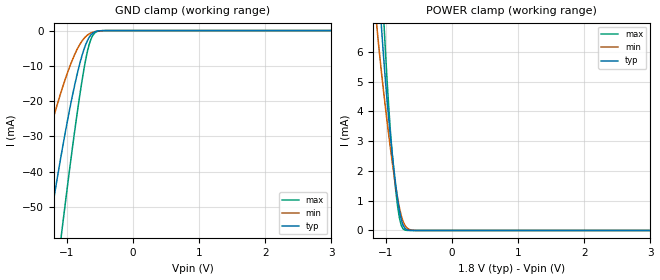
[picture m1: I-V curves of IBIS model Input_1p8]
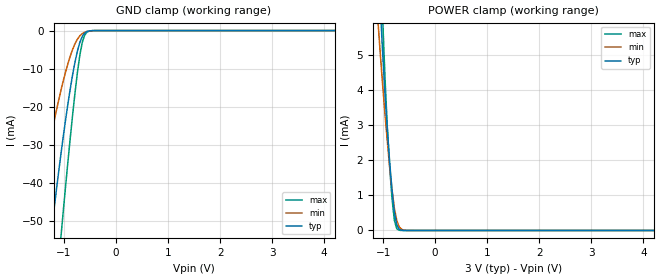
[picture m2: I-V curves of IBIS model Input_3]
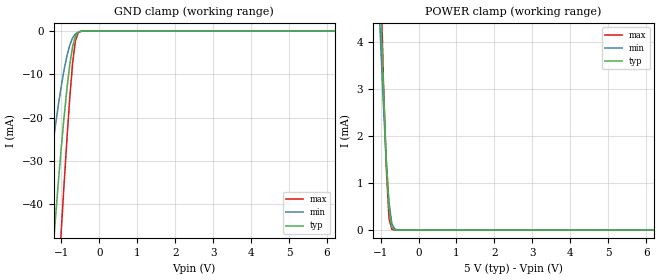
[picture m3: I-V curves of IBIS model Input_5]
|Texas Instruments Incorporated
|18-bit, Single Channgel, Low-Noise, Voltage-Output
|DIGITAL-TO-ANALOG CONVERTER
| Marketing part#   Voltage Range   Package-type   #pins
|DAC9881SBRGER   1.7V - 5V   VQFN   24-pin RGE
|DAC9881SBRGERG4   1.7V - 5V   VQFN   24-pin RGE
|DAC9881SBRGET   1.7V - 5V   VQFN   24-pin RGE
|DAC9881SBRGETG4   1.7V - 5V   VQFN   24-pin RGE
|DAC9881SRGER   1.7V - 5V   VQFN   24-pin RGE
|DAC9881SRGERG4   1.7V - 5V   VQFN   24-pin RGE
|DAC9881SRGET   1.7V - 5V   VQFN   24-pin RGE
|DAC9881SRGETG4   1.7V - 5V   VQFN   24-pin RGE
[IBIS Ver]   4.0
[File name]   dac9881a.ibs
[File Rev]   1.0
[Date]   07/08/2009
[Source]   Texas Instruments Incorporated.
   Analog-eLab, HPA
   12500 TI Blvd
   Dallas, TX -75243
   For Support e-mail: elab_ibis@list.ti.com
[Notes]   Revision History:
   1.0: 07/08/2009
   - Initial Model generated from simulations in TISPICED
   - Model not matched to measurements
   - Ignore warnings related to ccomp min max values, these are
   as per simulations in TISPICED, part uses BJT devices
[Disclaimer]
 This product is designed as an aid for customers of Texas Instruments.
 No warranties, either expressed or implied, with respect to this third
 party software (if any) or with respect to its fitness for any
 particular purpose is claimed by Texas Instruments or the author. The
 software (if any) is provided solely on an "as is" basis. The entire
 risk as to its quality and performance is with the customer
[Copyright] (C) Copyright 2009 Texas Instruments Incorporated.
   All rights reserved.
|   DAC9881A
[Component]   DAC9881A
[Manufacturer]  Texas Instruments Incorporated
[Package]   |24-pin RGE, VQFN 4mm X 4mm
|   typ   min   max
R_pkg   71.83m   62.81m   80.84m
L_pkg   1.169nH   1.006nH   1.332nH
C_pkg   0.103pF   0.094pF   0.112pF
[Pin]   signal_name   model_name   R_pin   L_pin   C_pin
   1   SCLK   Input   0.07599  1.23841nH   0.10623pF
   2   SDI   Input   0.07182  1.16214nH   0.10564pF
   3   LDAC#   Input   0.07043  1.13785nH   0.10439pF
   4   AGND   GND   0.03576  0.79035nH   0.14259pF
   5   AVDD   POWER   0.07196  1.16684nH   0.10654pF
   6   VREFLS   NC   0.07706  1.26253nH   0.10829pF
   7   VREFHS   NC   0.07013  1.13811nH   0.10024pF
   8   VOUT   NC   0.06281  1.00570nH   0.09441pF
   9   RFB   NC   0.06661  1.07325nH   0.10032pF
   10   VREFLF   NC   0.03298  0.69750nH   0.14107pF
   11   VREFHF   NC   0.03275  0.70664nH   0.14010pF
   12   NC   NC   0.07739  1.27043nH   0.11226pF
   13   NC   NC   0.08084  1.33221nH   0.11195pF
   14   RSTSEL   Input   0.07657  1.25184nH   0.11077pF
   15   GAIN   Input   0.07212  1.16965nH   0.10607pF
   16   USB_BTC#   Input   0.07043  1.13795nH   0.10403pF
   17   RST#   Input   0.07196  1.16454nH   0.10595pF
   18   PDN   Input   0.07653  1.24823nH   0.10633pF
   19   CS#   Input   0.07679  1.25161nH   0.10889pF
   20   SDOSEL   Input   0.06908  1.10924nH   0.10603pF
   21   AVDD   POWER   0.06763  1.08295nH   0.10070pF
   22   DGND   GND   0.06770  1.08415nH   0.09968pF
   23   SDO   Output   0.06834  1.09604nH   0.10367pF
   24   IOVDD   POWER   0.07464  1.21210nH   0.10622pF
|   25   NC   NC   0.00089  0.24393nH  1.30974pF  ||mountpad
[Model Selector]   Input
Input_1p8   IOVDD varies between 1.7V - 2.0V, typ value being 1.8V
Input_3   IOVDD varies between 2.7V - 3.3V, typ value being 3.0V
Input_5   IOVDD varies between 4.5V - 5.5V, typ value being 5.0V
[Model Selector]   Output
Output_1p8   IOVDD varies between 1.7V - 2.0V, typ value being 1.8V
Output_3   IOVDD varies between 2.7V - 3.3V, typ value being 3.0V
Output_5   IOVDD varies between 4.5V - 5.5V, typ value being 5.0V
| Models and submodels in the file (6): Input_1p8 (Input), Input_3 (Input), Input_5 (Input), Output_1p8 (3-state), Output_3 (3-state), Output_5 (3-state)
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|   Input 1.8V IOVDD
[Model]   Input_1p8
Model_type   Input
|Signals
|Input Levels
Vinl = 0V
Vinh = 1.5V
|   typ   min   max
C_comp   3.032pF   3.426pF   2.439pF
[Model Spec]
Vinl   0V   -0.3V   0.3V
Vinh   1.9V   1.5V   2.3V
[Voltage Range]   1.8V   1.7V   2.0V
| Junction Temperature (Ambient temp is 25C typ, 85C min,  -40C max)
[Temperature Range]   27.0   105.0   -40.0
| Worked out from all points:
|   GND clamp passes 1 mA (typ) near -0.62 V on its own axis
|   POWER clamp passes 1 mA (typ) near -0.82 V on its own axis
[GND Clamp]
|   Voltage   I(typ)   I(min)   I(max)
-1.8V     -124.5mA   -72.43mA   -174.7mA
-1.61V    -99.18mA   -55.82mA   -143.3mA
-1.284V   -58.12mA   -30.4mA    -90.01mA
-1.257V   -54.89mA   -28.5mA    -85.65mA
-1.067V   -33.54mA   -16.32mA   -55.8mA
-931.7mV  -20.04mA   -9.093mA   -35.69mA
-823.1mV  -10.85mA   -4.6mA     -20.89mA
-741.7mV  -5.439mA   -2.278mA   -11.1mA
-660.3mV  -1.897mA   -933.9uA   -3.886mA
-578.9mV  -387.6uA   -321.7uA   -706.2uA
-470.4mV  -25.45uA   -52.46uA   -29.69uA
3.6V      0A         0A         0A
[POWER Clamp]
|   Voltage   I(typ)   I(min)   I(max)
-1.8V     36.64mA    28.31mA    45.65mA
-1.149V   9.666mA    7.122mA    12.38mA
-1.122V   8.678mA    6.481mA    11.09mA
-1.067V   6.82mA     5.306mA    8.583mA
-1.04V    5.967mA    4.76mA     7.384mA
-1.013V   5.177mA    4.233mA    6.238mA
-931.7mV  3.15mA     2.753mA    3.312mA
-850.3mV  1.504mA    1.451mA    1.307mA
-796mV    664.8uA    761.1uA    419.8uA
-714.6mV  74.74uA    176.1uA    16.51uA
-524.6mV  78.53nA    1.039uA    4.643nA
3.6V      0A         0A         0A
|   Input 3.0V IOVDD
[Model]   Input_3
Model_type   Input
Vinl = 0.15V
Vinh = 2.85V
|   typ   min   max
C_comp   2.779pF   3.181pF   2.237pF
[Model Spec]
Vinl   0.15V   -0.3V   0.6V
Vinh   2.85V   2.1V   3.6V
[Voltage Range]   3.000V   2.700V   3.300V
| Junction Temperature (Ambient temp is 25C typ, 105C min,  -40C max)
[Temperature Range]   27.0   105.0   -40.0
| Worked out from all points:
|   GND clamp passes 1 mA (typ) near -0.62 V on its own axis
|   POWER clamp passes 1 mA (typ) near -0.82 V on its own axis
[GND Clamp]
|   Voltage   I(typ)   I(min)   I(max)
-3V       -292.7mA   -193.9mA   -373.2mA
-1.598V   -97.6mA    -54.8mA    -141.3mA
-1.553V   -91.7mA    -51.04mA   -133.8mA
-1.236V   -52.41mA   -27.04mA   -82.27mA
-1.055V   -32.27mA   -15.62mA   -53.96mA
-1.01V    -27.62mA   -13.09mA   -47.15mA
-874.4mV  -14.97mA   -6.547mA   -27.69mA
-738.7mV  -5.271mA   -2.211mA   -10.78mA
-648.2mV  -1.554mA   -806.3uA   -3.158mA
-603mV    -656.4uA   -449.5uA   -1.26mA
-422.1mV  -6.58uA    -17.45uA   -5.716uA
6V        0A         0A         0A
[POWER Clamp]
|   Voltage   I(typ)   I(min)   I(max)
-3V       88.98mA    71.68mA    109mA
-1.101V   7.934mA    6.009mA    10.1mA
-1.055V   6.434mA    5.06mA     8.045mA
-1.01V    5.093mA    4.176mA    6.115mA
-919.6mV  2.885mA    2.546mA    2.962mA
-874.4mV  1.954mA    1.811mA    1.821mA
-829.1mV  1.145mA    1.16mA     911uA
-783.9mV  521.9uA    637.3uA    291.2uA
-738.7mV  162.6uA    289.1uA    49.37uA
-693.5mV  35.79uA    110uA      6.239uA
-512.6mV  51.38nA    729.5nA    2.907nA
6V        0A         0A         0A
|   Input 5.0V IOVDD
[Model]   Input_5
Model_type   Input
Vinl = 0.25V
Vinh = 4.55V
|   typ   min   max
C_comp   2.503pF   2.891pF   2.007pF
[Model Spec]
Vinl   0.25V   -0.3V   0.8V
Vinh   4.55V   3.8V   5.3V
[Voltage Range]   5.000V   4.500V   5.500V
| Junction Temperature (Ambient temp is 25C typ, 105C min,  -40C max)
[Temperature Range]   27.0   105.0   -40.0
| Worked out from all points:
|   GND clamp passes 1 mA (typ) near -0.62 V on its own axis
|   POWER clamp passes 1 mA (typ) near -0.82 V on its own axis
[GND Clamp]
|   Voltage   I(typ)   I(min)   I(max)
-5V       -578.6mA   -418.3mA   -700.9mA
-1.533V   -89.1mA    -49.39mA   -130.5mA
-1.457V   -79.45mA   -43.34mA   -118.1mA
-1.231V   -51.82mA   -26.7mA    -81.46mA
-1.156V   -43.19mA   -21.73mA   -69.52mA
-1.005V   -27.12mA   -12.82mA   -46.4mA
-854.3mV  -13.3mA    -5.743mA   -24.98mA
-778.9mV  -7.713mA   -3.214mA   -15.38mA
-703.5mV  -3.515mA   -1.534mA   -7.264mA
-628.1mV  -1.083mA   -626uA     -2.159mA
-552.8mV  -210.4uA   -219.4uA   -355.2uA
10V       0A         0A         0A
[POWER Clamp]
|   Voltage   I(typ)   I(min)   I(max)
-5V       176.5mA    144.7mA    214.3mA
-1.08V    7.25mA     5.578mA    9.175mA
-1.005V   4.954mA    4.081mA    5.912mA
-929.6mV  3.106mA    2.718mA    3.252mA
-854.3mV  1.577mA    1.509mA    1.388mA
-778.9mV  468uA      589.4uA    246.4uA
-703.5mV  51.06uA    138.2uA    9.916uA
-628.1mV  3.286uA    20.79uA    335nA
-477.4mV  15.16nA    260.7nA    830.6pA
10V       0A         0A         0A
